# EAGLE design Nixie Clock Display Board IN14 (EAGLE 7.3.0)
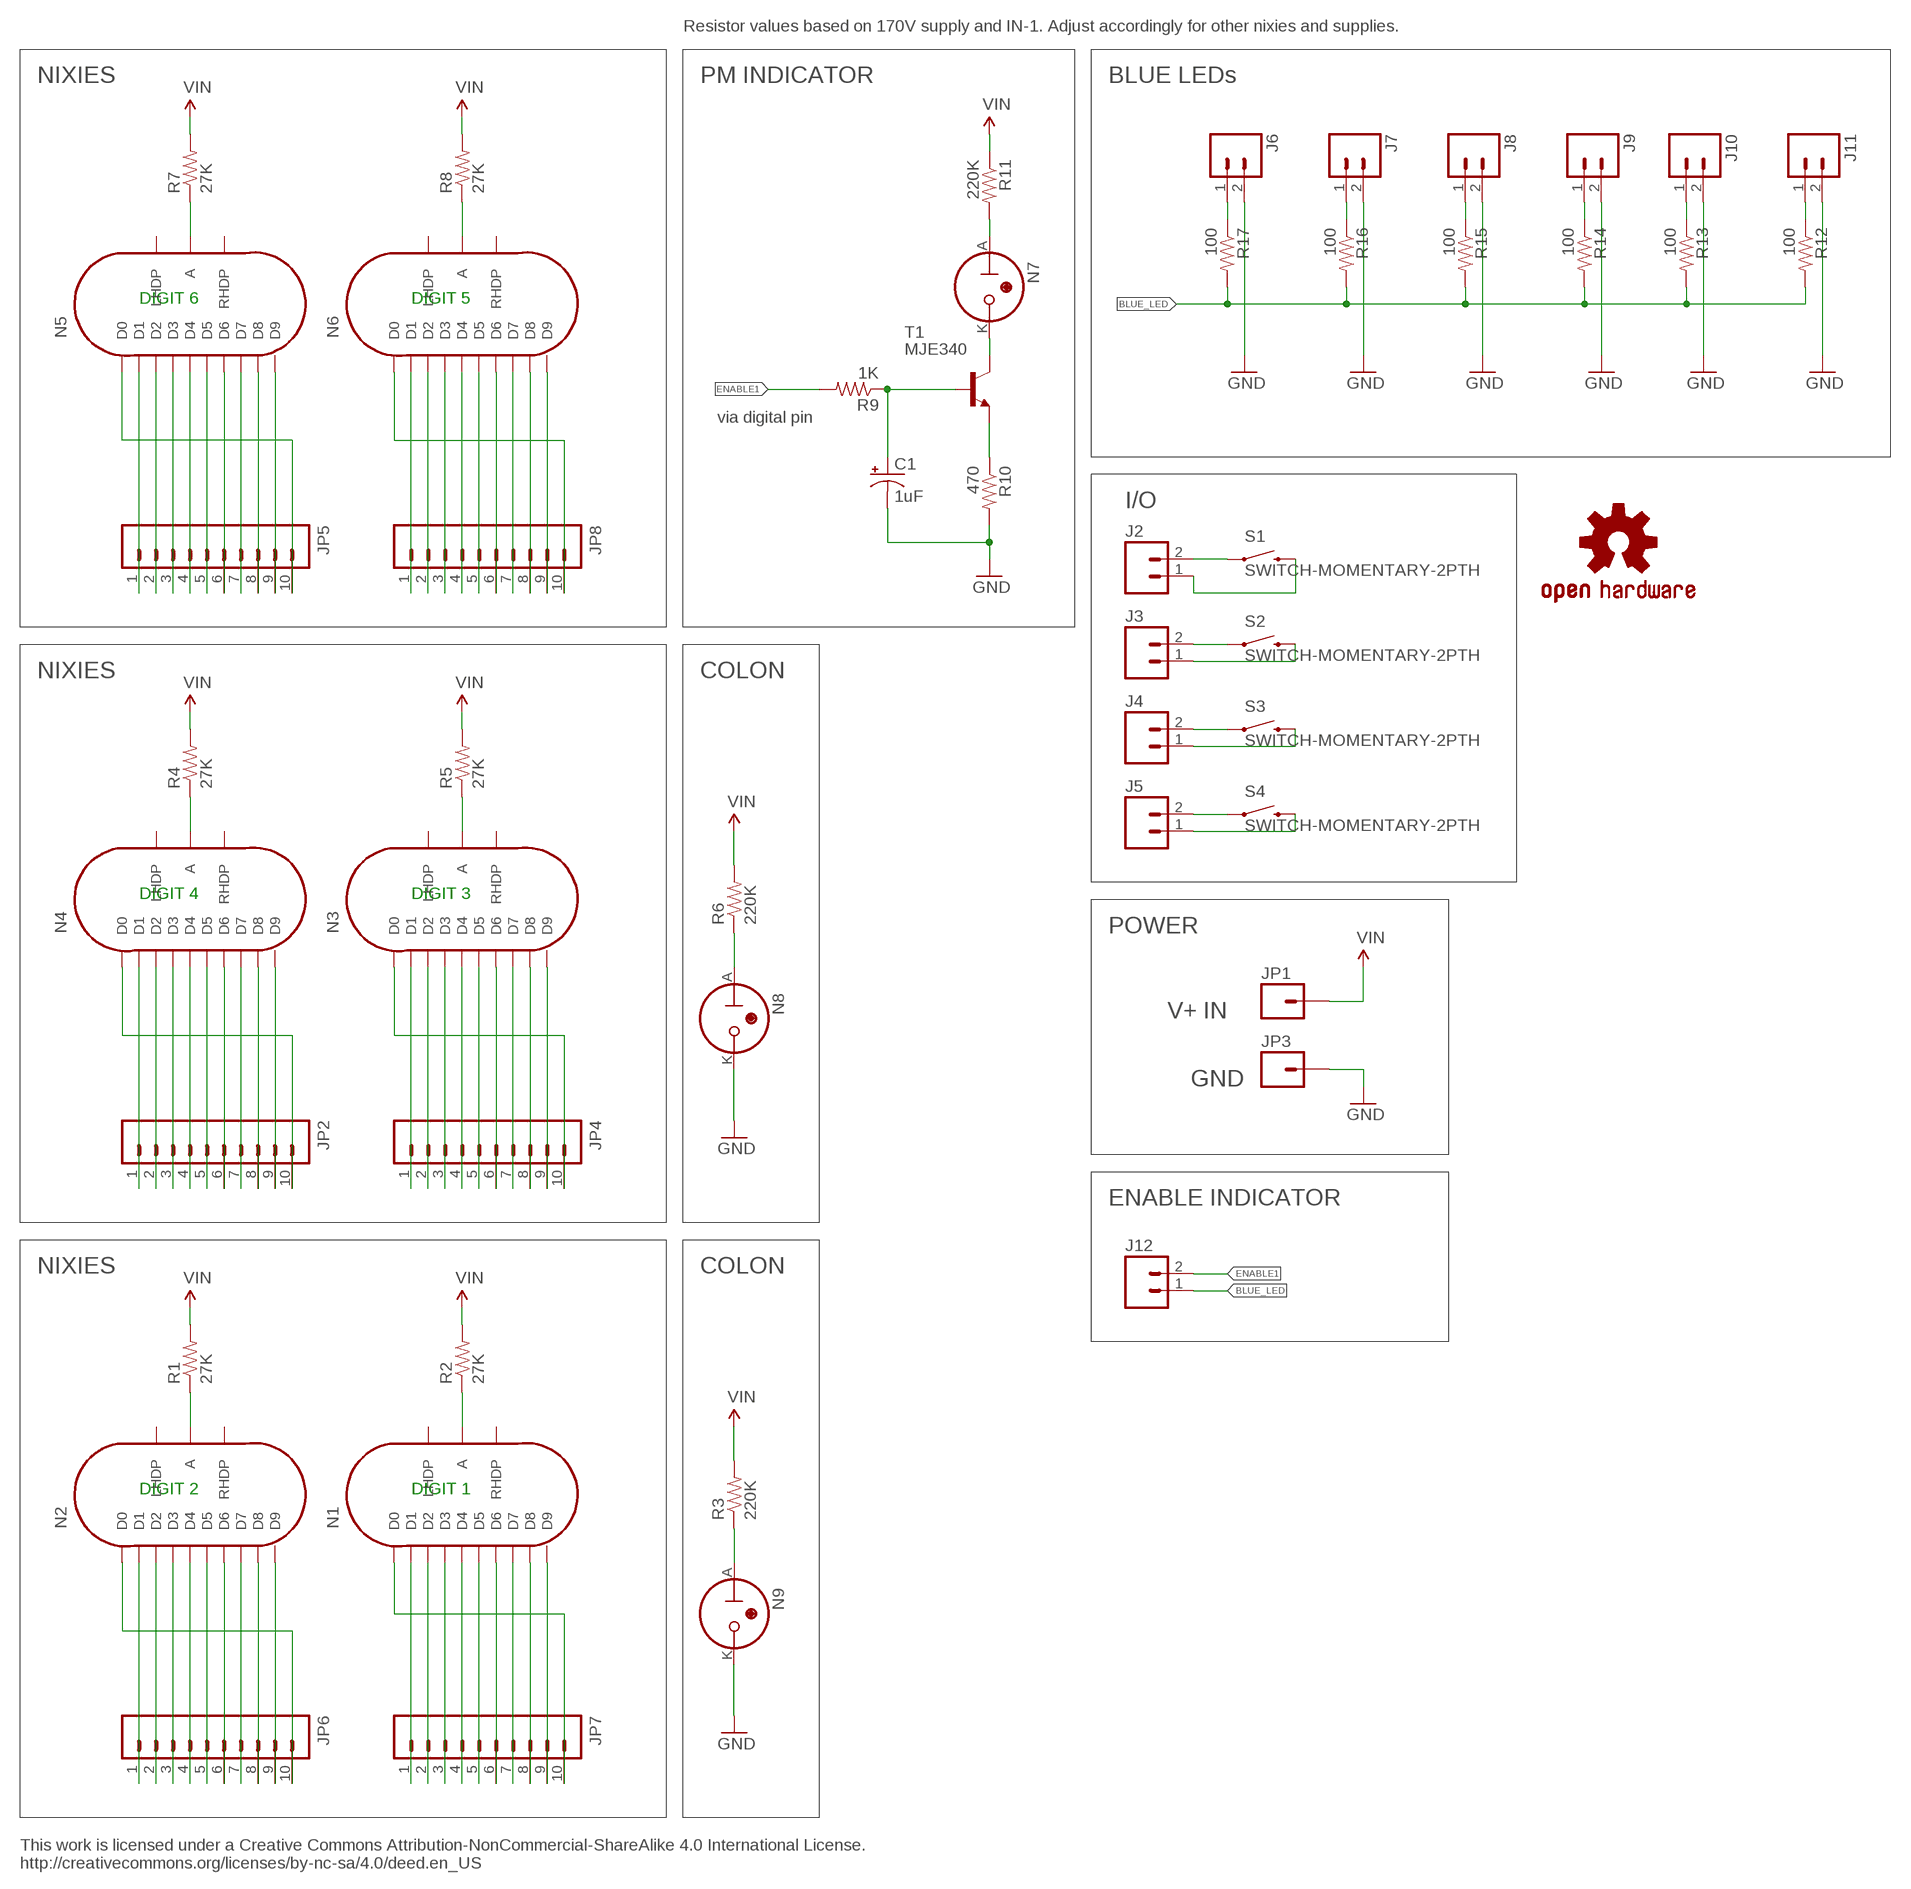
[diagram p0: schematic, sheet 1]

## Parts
C1  1uF  CAP_POLPTH2  [CPOL-RADIAL-10UF-25V]
J2  M02PTH  [1X02]
J3  M02PTH  [1X02]
J4  M02PTH  [1X02]
J5  M02PTH  [1X02]
J6  M02PTH  [1X02]
J7  M02PTH  [1X02]
J8  M02PTH  [1X02]
J9  M02PTH  [1X02]
J10  M02PTH  [1X02]
J11  M02PTH  [1X02]
J12  M02PTH  [1X02]
JP1  M01PTH  [1X01]
JP2  M10"  [1X10]
JP3  M01PTH  [1X01]
JP4  M10"  [1X10]
JP5  M10"  [1X10]
JP6  M10"  [1X10]
JP7  M10"  [1X10]
JP8  M10"  [1X10]
N1  IN-14  [IN-14]
N2  IN-14  [IN-14]
N3  IN-14  [IN-14]
N4  IN-14  [IN-14]
N5  IN-14  [IN-14]
N6  IN-14  [IN-14]
N7  IN-3  [IN-3]
N8  IN-3  [IN-3]
N9  IN-3  [IN-3]
R1  27K  RESISTORPTH-1/2W  [AXIAL-0.5]
R2  27K  RESISTORPTH-1/2W  [AXIAL-0.5]
R3  220K  RESISTORPTH-1/2W  [AXIAL-0.5]
R4  27K  RESISTORPTH-1/2W  [AXIAL-0.5]
R5  27K  RESISTORPTH-1/2W  [AXIAL-0.5]
R6  220K  RESISTORPTH-1/2W  [AXIAL-0.5]
R7  27K  RESISTORPTH-1/2W  [AXIAL-0.5]
R8  27K  RESISTORPTH-1/2W  [AXIAL-0.5]
R9  1K  RESISTORPTH-1/2W  [AXIAL-0.5]
R10  470  RESISTORPTH-1/2W  [AXIAL-0.5]
R11  220K  RESISTORPTH-1/2W  [AXIAL-0.5]
R12  100  RESISTOR0805-RES  [0805]
R13  100  RESISTOR0805-RES  [0805]
R14  100  RESISTOR0805-RES  [0805]
R15  100  RESISTOR0805-RES  [0805]
R16  100  RESISTOR0805-RES  [0805]
R17  100  RESISTOR0805-RES  [0805]
S1  SWITCH-MOMENTARY-2PTH  [TACTILE-PTH]
S2  SWITCH-MOMENTARY-2PTH  [TACTILE-PTH]
S3  SWITCH-MOMENTARY-2PTH  [TACTILE-PTH]
S4  SWITCH-MOMENTARY-2PTH  [TACTILE-PTH]
T1  MJE340  -NPN-TO225AA  [TO225AA]
U$2  OSHW-LOGOM  [OSHW-LOGO-M]

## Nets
BLUE_LED: J12.1 R12.2 R13.2 R14.2 R15.2 R16.2 R17.2
ENABLE1: J12.2 R9.P$2
GND: C1.2(-) J6.2 J7.2 J8.2 J9.2 J10.2 J11.2 JP3.1 N8.K N9.K R10.P$2
N$1: N8.A R6.P$1
N$4: J2.1 S1.3
N$5: J2.2 S1.1
N$6: J3.2 S2.1
N$7: JP2.6 N4.D6
N$8: JP2.9 N4.D9
N$9: JP2.8 N4.D8
N$10: JP2.10 N4.D0
N$11: JP2.7 N4.D7
N$12: JP2.5 N4.D5
N$13: JP2.4 N4.D4
N$14: JP2.3 N4.D3
N$15: JP2.2 N4.D2
N$16: JP2.1 N4.D1
N$17: JP4.6 N3.D6
N$18: JP4.9 N3.D9
N$19: JP4.8 N3.D8
N$20: JP4.10 N3.D0
N$21: J3.1 S2.3
N$22: C1.1(+) R9.P$1 T1.1(B)
N$23: N7.A R11.P$2
N$24: R10.P$1 T1.3(E)
N$25: JP4.7 N3.D7
N$26: JP4.5 N3.D5
N$27: J4.2 S3.1
N$28: N7.K T1.2(C)
N$29: N5.A R7.P$1
N$30: JP5.6 N5.D6
N$31: JP5.9 N5.D9
N$32: JP5.8 N5.D8
N$33: JP5.10 N5.D0
N$34: JP5.7 N5.D7
N$35: JP5.5 N5.D5
N$36: JP5.4 N5.D4
N$37: JP5.3 N5.D3
N$38: JP5.2 N5.D2
N$39: JP5.1 N5.D1
N$40: N6.A R8.P$1
N$41: JP8.6 N6.D6
N$42: JP8.9 N6.D9
N$43: JP8.8 N6.D8
N$44: JP8.10 N6.D0
N$45: JP8.7 N6.D7
N$46: JP8.5 N6.D5
N$47: JP8.4 N6.D4
N$48: JP8.3 N6.D3
N$49: JP8.2 N6.D2
N$50: JP8.1 N6.D1
N$51: JP4.4 N3.D4
N$52: JP4.3 N3.D3
N$53: JP4.2 N3.D2
N$54: JP4.1 N3.D1
N$55: N4.A R4.P$1
N$56: N3.A R5.P$1
N$57: N9.A R3.P$1
N$58: J4.1 S3.3
N$59: J5.2 S4.1
N$60: J5.1 S4.3
N$62: J6.1 R17.1
N$63: JP6.6 N2.D6
N$64: JP6.9 N2.D9
N$65: JP6.8 N2.D8
N$66: JP6.10 N2.D0
N$67: JP6.7 N2.D7
N$68: JP6.5 N2.D5
N$69: JP6.4 N2.D4
N$70: JP6.3 N2.D3
N$71: JP6.2 N2.D2
N$72: JP6.1 N2.D1
N$73: JP7.6 N1.D6
N$74: JP7.9 N1.D9
N$75: JP7.8 N1.D8
N$76: JP7.10 N1.D0
N$77: JP7.7 N1.D7
N$78: JP7.5 N1.D5
N$79: JP7.4 N1.D4
N$80: JP7.3 N1.D3
N$81: JP7.2 N1.D2
N$82: JP7.1 N1.D1
N$83: N2.A R1.P$1
N$84: N1.A R2.P$1
N$87: J7.1 R16.1
N$90: J8.1 R15.1
N$93: J9.1 R14.1
N$96: J10.1 R13.1
N$99: J11.1 R12.1
VIN: JP1.1 R1.P$2 R2.P$2 R3.P$2 R4.P$2 R5.P$2 R6.P$2 R7.P$2 R8.P$2 R11.P$1
Unconnected: N1.LHDP N1.RHDP N2.LHDP N2.RHDP N3.LHDP N3.RHDP N4.LHDP N4.RHDP N5.LHDP N5.RHDP N6.LHDP N6.RHDP

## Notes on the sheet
- Resistor values based on 170V supply and IN-1. Adjust accordingly for other nixies and supplies.
- NIXIES | PM INDICATOR | BLUE LEDs
- DIGIT 6 | DIGIT 5
- via digital pin
- I/O
- NIXIES | COLON
- DIGIT 4 | DIGIT 3
- POWER
- V+ IN
- GND
- ENABLE INDICATOR
- NIXIES | COLON
- DIGIT 2 | DIGIT 1
- This work is licensed under a Creative Commons Attribution-NonCommercial-ShareAlike 4.0 International License.
  http://creativecommons.org/licenses/by-nc-sa/4.0/deed.en_US

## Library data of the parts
C1 = SparkFun-Capacitors:CAP_POL: Capacitor Polarized
J2-J12 = SparkFun-Connectors:M02: Standard 2-pin 0.1" header. Use with
JP1 JP3 = SparkFun-Connectors:M01: Header 1
JP2 JP4-JP8 = SparkFun-Connectors:M10: Header 10 Standard 10-pin 0.1" header. Use with straight break away headers (SKU : PRT-00116), right angle break away headers (PRT-00553), swiss pins (PRT-00743), machine pins (PRT-00117), and female headers (PRT-00115).
N1-N6 = russian-nixies:IN-14: IN-14: medium numeric frontview nixie tube
N7-N9 = Nixie Tubes 2:IN-3: IN-3: nixie bulb
R1-R17 = SparkFun-Resistors:RESISTOR: Resistor
S1-S4 = SparkFun-Electromechanical:SWITCH-MOMENTARY-2: Various NO switches- pushbuttons, reed, etc; PROD_ID: SWCH-08441
T1 = Transistor 2:*-NPN-: NPN Transistror BF959 corrected 2008.03.06
U$2 = SparkFun:OSHW-LOGO: Open Source Hardware Logo This logo indicates the piece of hardware it is found on incorporates a OSHW license and/or adheres to the definition of open source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

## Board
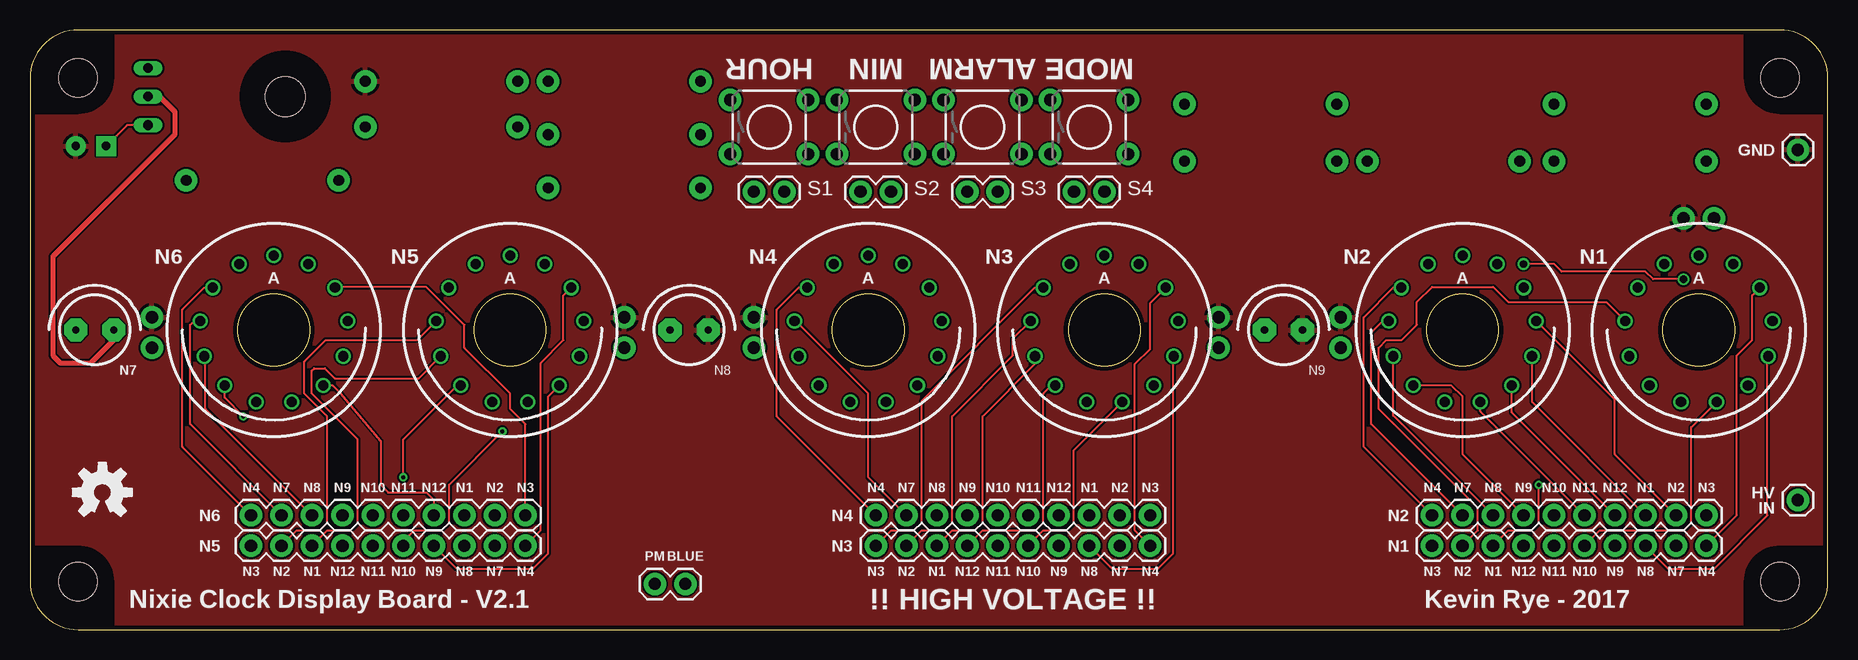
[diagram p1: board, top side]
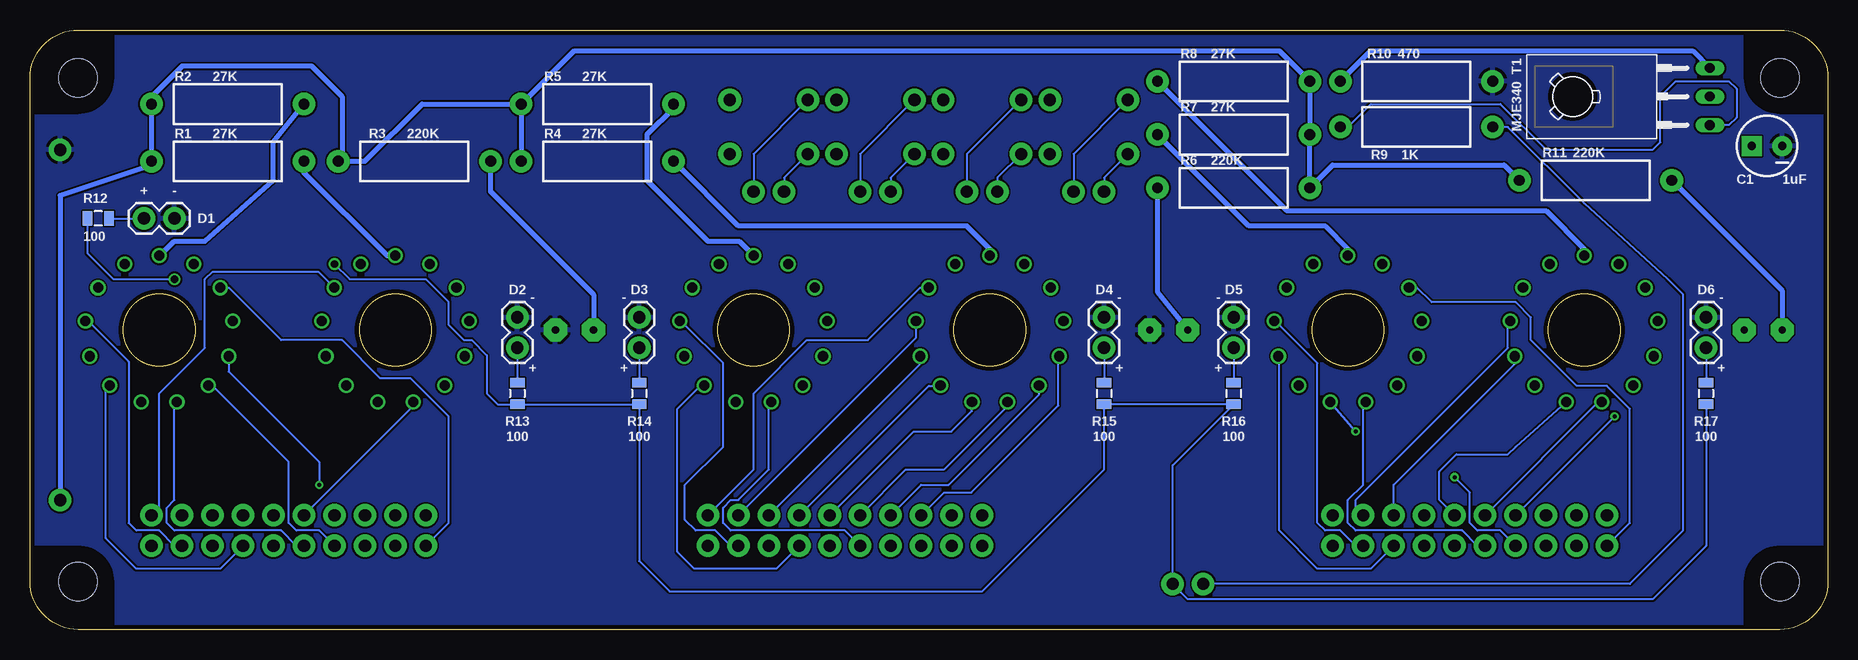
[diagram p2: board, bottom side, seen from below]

Size 149.83 x 50 mm. Coordinates in mm from the lower left corner, seen from the top.
Outline: circle at 20.32,24.99 radius 3
Outline: circle at 40.01,24.99 radius 3
Outline: circle at 69.85,24.99 radius 3
Outline: circle at 89.53,24.99 radius 3
Outline: circle at 119.38,24.99 radius 3
Outline: circle at 139.06,24.99 radius 3
Copper layers (1*16): Top 0.0356mm / dielectric 1.5011mm / Bottom 0.0356mm
Design rules "LaenPCBOrder": minimum track width 6mil, minimum drill 13mil, track to track 6mil, track to pad 6mil, pad to pad 6mil, via to via 6mil, smd to smd 6mil, copper to edge 15mil, drill to drill 6mil, minimum pad ring 7mil, minimum via ring 7mil, stop-mask expansion 3mil, vias tented up to drill 0mil, thermal gap 10mil

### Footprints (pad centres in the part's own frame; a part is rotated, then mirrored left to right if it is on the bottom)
CPOL-RADIAL-10UF-25V = drill 0.7 pad 1.651 square: 1 1.27,0 | drill 0.7 pad 1.651: 2 -1.27,0
1X02 = drill 1.016 pad 1.88: 1 0,0; 2 2.54,0
1X01 = drill 1.016 pad 1.88: 1 0,0
1X10 = drill 1.016 pad 1.88: 1 0,0; 2 2.54,0; 3 5.08,0; 4 7.62,0; 5 10.16,0; 6 12.7,0; 7 15.24,0; 8 17.78,0; 9 20.32,0; 10 22.86,0
IN-14 = drill 0.84: A 0,-6.19; D0 -5.094,-3.516; D1 5.094,-3.516; D2 6.145,-0.746; D3 5.788,2.195; D4 4.105,4.633; D5 1.481,6.01; D6 -1.481,6.01; D7 -4.105,4.633; D8 -5.788,2.195; D9 -6.145,-0.746; LHDP 2.877,-5.481; RHDP -2.877,-5.481
IN-3 = drill 0.6 pad 1.93 octagon: A -1.587,0; K 1.587,0
AXIAL-0.5 = drill 0.9 pad 1.88: P$1 -6.35,0; P$2 6.35,0
0805 = smd 0.8 x 1.2: 1 -0.9,0; 2 0.9,0
TACTILE-PTH = drill 1.016 pad 1.88: 1 -3.251,2.261; 2 3.251,2.261; 3 -3.251,-2.261; 4 3.251,-2.261
TO225AA = drill 0.813 long: 1 -2.381,-11.43; 2 0,-11.43; 3 2.381,-11.43 | hole 3.302: 0,0
50X150 = hole 3.2: 4,4; 145.83,4; 145.83,46; 4,46

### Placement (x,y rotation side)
C1  5.08,40.32 180 bottom
J2  60.33,36.51 0 top
J3  69.22,36.51 0 top
J4  78.11,36.51 0 top
J5  87,36.51 0 top
J6  10.16,23.5 90 bottom
J7  49.53,23.5 90 bottom
J8  60.33,23.5 90 bottom
J9  99.06,23.5 90 bottom
J10  109.22,23.5 90 bottom
J11  140.34,34.29 0 bottom
J12  54.61,3.81 180 top
JP1  147.32,10.79 0 top
JP2  70.48,9.53 0 top
JP3  147.32,40.01 0 top
JP4  70.48,6.99 0 top
JP5  18.41,6.99 0 top
JP6  116.84,9.53 0 top
JP7  116.84,6.99 0 top
JP8  18.41,9.53 0 top
N1  139.06,24.99 180 top
N2  119.38,24.99 180 top
N3  89.53,24.99 180 top
N4  69.85,24.99 180 top
N5  40.01,24.99 180 top
N6  20.32,24.99 180 top
N7  5.4,24.99 0 top
N8  54.93,24.99 0 top
N9  104.46,24.99 0 top
R1  133.35,39.05 180 bottom
R2  133.35,43.81 180 bottom
R3  117.79,39.05 180 bottom
R4  102.55,39.05 180 bottom
R5  102.55,43.81 180 bottom
R6  49.53,36.83 0 bottom
R7  49.53,41.27 0 bottom
R8  49.53,45.72 0 bottom
R9  34.29,41.91 0 bottom
R10  34.29,45.72 0 bottom
R11  19.37,37.47 0 bottom
R12  144.15,34.29 180 bottom
R13  109.22,19.68 270 bottom
R14  99.06,19.68 270 bottom
R15  60.33,19.68 270 bottom
R16  49.53,19.68 270 bottom
R17  10.16,19.68 270 bottom
S1  61.59,41.91 0 top
S2  70.48,41.91 0 top
S3  79.38,41.91 0 top
S4  88.27,41.91 0 top
T1  21.27,44.45 90 bottom
U$1  [50X150]  0,0 0 top
U$2  6.03,11.43 0 top

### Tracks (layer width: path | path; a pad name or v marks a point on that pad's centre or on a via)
BLUE_LED  (via drill 0.61)
  Top 0.152: v137.79,29.21 135.25,29.21 134.62,29.84 127.64,29.84 127,30.48 v124.46,30.48
  Bottom 0.152: R17.2 10.16,6.99 14.61,2.54 53.34,2.54 J12.1 54.61,13.71 R16.2 R15.2 60.33,13.34 70.48,3.17 96.52,3.17 99.06,5.71 R14.2 R13.2 110.86,18.79 111.76,19.68 111.76,22.86 113.03,24.13 113.67,24.13 114.94,25.4 114.94,27.3 116.84,29.21 123.19,29.21 v124.46,30.48 | R12.2 145.04,31.38 142.88,29.21 v137.79,29.21
ENABLE1
  Bottom 0.152: R9.P$2 26.67,41.91 20.32,35.56 13.34,29.21 12.06,27.94 12.06,8.26 16.51,3.81 J12.2
GND
  pour Bottom: -0.64,50.8 150.5,50.8 150.5,-0.64 -0.64,-0.64
  pour Top: -1.27,51.44 151.13,51.44 151.13,-1.27 -1.27,-1.27
N$1
  Bottom 0.406: R6.P$1 55.88,28.16 N8.A
N$4
  Bottom 0.152: S1.3 60.33,37.67 J2.1
N$5
  Bottom 0.152: S1.1 62.87,39.65 J2.2
N$6
  Bottom 0.152: S2.1 71.75,39.65 J3.2
N$7
  Bottom 0.152: JP2.6 76.2,16.51 73.04,16.51 71.33,18.22 N4.D6
N$8
  Bottom 0.152: JP2.9 76,24.34 N4.D9
N$9
  Bottom 0.152: JP2.8 75.64,22.15 N4.D8
N$10
  Bottom 0.152: JP2.10 89.53,13.34 89.53,19.68 85.09,24.13 80.01,24.13 75.64,28.5 N4.D0
N$11
  Bottom 0.152: JP2.7 74.93,20.32 74.3,20.32 N4.D7
N$12
  Bottom 0.152: JP2.5 76.83,13.34 73.66,13.34 68.37,18.63 N4.D5
N$13
  Bottom 0.152: JP2.4 75.56,12.06 73.28,12.06 65.75,19.6 N4.D4
N$14
  Bottom 0.152: JP2.3 73.66,11.43 71.38,11.43 64.14,18.67 64.14,22.23 N4.D3
N$15
  Top 0.152: JP2.2 69.85,12.7 69.85,19.68 63.8,25.73 N4.D2
N$16
  Top 0.152: JP2.1 62.23,17.78 62.23,26.67 64.06,28.5 N4.D1
N$17
  Top 0.152: JP4.6 84.45,8.26 86.36,8.26 87,8.89 87,14.96 N3.D6
N$18
  Bottom 0.152: JP4.9 91.44,6.99 92.71,8.26 94.35,8.26 95.25,9.15 95.25,12.06 92.08,15.24 92.08,22.23 95.25,25.4 N3.D9
N$19
  Top 0.152: JP4.8 90.17,5.08 93.98,5.08 95.25,6.35 95.25,22.72 N3.D8
N$20
  Top 0.152: JP4.10 92.08,8.26 92.08,22.14 93.34,23.41 93.34,27.22 N3.D0
N$21
  Bottom 0.152: S2.3 69.22,37.67 J3.1
N$22
  Top 0.152: T1.1 8.1,42.07 C1.1
  Bottom 0.152: R9.P$1 40.01,41.91 38.1,43.81 27.3,43.81 23.5,40.01 14.61,40.01 13.97,40.64 13.97,44.45 12.7,45.72 8.26,45.72 7.62,45.09 7.62,42.7 8.26,42.07 T1.1
N$23
  Bottom 0.406: R11.P$2 3.81,28.26 N7.A
N$24
  Bottom 0.406: R10.P$1 38.1,48.26 11.27,48.26 T1.3
N$25
  Bottom 0.152: JP4.7 87.63,5.08 94.47,5.08 95.89,6.5 95.89,18.41 93.98,20.32 N3.D7
N$26
  Bottom 0.152: JP4.5 81.92,8.26 91.44,8.26 92.08,8.89 92.08,10.16 91.44,10.79 90.81,10.79 88.27,13.34 88.27,18.41 N3.D5
N$27
  Bottom 0.152: S3.1 80.64,39.65 J4.2
N$28
  Top 0.406: T1.2 10.79,44.45 12.06,43.18 12.06,41.27 1.91,31.11 1.91,22.86 2.54,22.23 5.08,22.23 6.99,24.13 N7.K
N$29
  Bottom 0.406: N5.A 40.01,31.75 41.91,33.66 48.26,33.66 R7.P$1
N$30  (via drill 0.33)
  Top 0.152: v39.37,16.51 34.92,12.06 34.92,8.89 34.29,8.26 32.01,8.26 31.11,7.36 JP5.6
  Bottom 0.152: v39.37,16.51 N5.D6
N$31
  Bottom 0.152: JP5.9 39.37,6.99 40.64,8.26 41.91,8.26 42.55,8.89 42.55,22.23 45.72,25.4 N5.D9
N$32
  Bottom 0.152: JP5.8 38.1,5.08 42.55,5.08 45.72,8.26 45.72,22.23 N5.D8
N$33
  Top 0.152: JP5.10 42.55,8.26 42.55,22.23 44.45,24.13 44.45,27.85 N5.D0
N$34
  Top 0.152: JP5.7 35.56,5.08 41.91,5.08 43.18,6.35 43.18,19.42 N5.D7
N$35
  Bottom 0.152: JP5.5 29.21,6.99 30.48,8.26 39.37,8.26 40.01,8.89 40.01,10.79 38.73,12.06 38.73,18.41 N5.D5
N$36  (via drill 0.33)
  Top 0.152: v31.11,12.7 31.11,15.88 35.59,20.35 N5.D4
  Bottom 0.152: v31.11,12.7 29.84,11.43 29.84,8.89 29.21,8.26 27.3,8.26 JP5.4
N$37
  Top 0.152: JP5.3 24.77,8.26 26.67,8.26 27.3,8.89 27.3,15.88 23.5,19.68 23.5,21.59 23.68,21.78 24.58,21.78 25.4,20.95 32.38,20.95 N5.D3
N$38
  Top 0.152: JP5.2 22.23,8.26 24.13,8.26 24.77,8.89 24.77,17.78 22.86,19.68 22.86,22.33 24.66,24.13 32.26,24.13 N5.D2
N$39
  Bottom 0.152: JP5.1 16.51,8.89 16.51,18.41 18.41,20.32 20.95,20.32 24.77,24.13 24.77,26.04 26.04,27.3 33.02,27.3 34.29,28.57 N5.D1
N$40
  Bottom 0.406: N6.A 20.32,31.75 23.5,34.92 45.09,34.92 R8.P$1
N$41
  Bottom 0.152: JP8.6 32.38,10.79 32.38,13.19 30.96,14.61 26.67,14.61 26.04,15.24 N6.D6
N$42
  Bottom 0.152: JP8.9 39.37,9.53 39.37,10.79 26.67,23.5 26.67,25.4 N6.D9
N$43
  Bottom 0.152: JP8.8 36.2,12.06 26.04,22.23 N6.D8
N$44
  Top 0.152: JP8.10 41.27,17.14 40.01,18.41 40.01,19.68 36.2,23.5 36.2,25.4 33.02,28.57 26.04,28.57 N6.D0
N$45
  Top 0.152: JP8.7 33.66,10.79 33.02,11.43 29.84,11.43 29.21,12.06 29.21,15.74 25.9,19.68 25.23,20.35 N6.D7
N$46
  Bottom 0.152: JP8.5 19.12,18.98 N6.D5
N$47  (via drill 0.33)
  Top 0.152: v17.78,17.78 16.21,19.34 N6.D4
  Bottom 0.152: JP8.4 v17.78,17.78
N$48
  Top 0.152: JP8.3 14.61,18.41 14.61,22.23 N6.D3
N$49
  Top 0.152: JP8.2 13.34,17.14 13.34,25.4 13.67,25.73 N6.D2
N$50
  Top 0.152: JP8.1 12.7,15.24 12.7,26.67 14.53,28.5 N6.D1
N$51
  Top 0.152: JP4.4 79.38,8.26 83.82,8.26 84.45,8.89 84.45,19.68 85.12,20.35 N3.D4
N$52
  Top 0.152: JP4.3 76.83,8.26 78.74,8.26 79.38,8.89 79.38,17.78 83.75,22.15 N3.D3
N$53
  Top 0.152: JP4.2 74.3,8.26 76.2,8.26 76.83,8.89 76.83,17.78 81.92,22.86 81.92,24.26 N3.D2
N$54
  Top 0.152: JP4.1 71.75,8.26 73.66,8.26 74.3,8.89 74.3,19.05 83.75,28.5 N3.D1
N$55
  Bottom 0.406: N4.A 69.85,31.75 71.75,33.66 90.81,33.66 R4.P$1
N$56
  Bottom 0.406: R5.P$1 96.2,43.5 98.42,41.27 98.42,37.47 93.34,32.38 90.74,32.38 N3.A
N$57
  Bottom 0.406: N9.A 102.87,27.94 111.44,36.51 R3.P$1
N$58
  Bottom 0.152: S3.3 78.11,37.67 J4.1
N$59
  Bottom 0.152: S4.1 89.53,39.65 J5.2
N$60
  Bottom 0.152: S4.3 87,37.67 J5.1
N$62
  Bottom 0.152: J6.1 R17.1
N$63
  Top 0.152: JP6.6 120.86,18.2 N2.D6
N$64
  Top 0.152: JP6.9 132.08,14.61 132.08,19.18 N2.D9
N$65
  Top 0.152: JP6.8 125.17,18.98 N2.D8
N$66
  Bottom 0.152: JP6.10 139.06,10.16 139.06,19.68 135.25,23.5 135.25,29.21 134.62,29.84 125.82,29.84 N2.D0
N$67
  Top 0.152: JP6.7 123.48,18.12 N2.D7
N$68
  Bottom 0.152: JP6.5 117.9,18.63 N2.D5
N$69
  Top 0.152: JP6.4 119.38,14.61 119.38,19.42 118.45,20.35 N2.D4
N$70
  Top 0.152: JP6.3 113.59,17.85 N2.D3
N$71
  Top 0.152: JP6.2 111.76,17.14 111.76,24.77 112.73,25.73 N2.D2
N$72
  Top 0.152: JP6.1 111.12,15.24 111.12,26.04 113.59,28.5 N2.D1
N$73
  Top 0.152: JP7.6 130.81,8.26 137.79,8.26 138.43,8.89 138.43,16.86 N1.D6
N$74
  Bottom 0.152: N1.D9 144.99,25.73 141.6,22.35 141.6,8.89 140.97,8.26 139.06,8.26 137.79,6.99 JP7.9
N$75
  Top 0.152: JP7.8 136.53,5.08 140.34,5.08 144.78,9.53 144.78,22.72 N1.D8
N$76
  Top 0.152: JP7.10 142.24,9.53 142.24,22.86 143.51,24.13 143.51,27.85 N1.D0
N$77
  Bottom 0.152: JP7.7 133.99,5.08 140.97,5.08 143.51,7.62 143.51,20.01 N1.D7
N$78
  Bottom 0.152: JP7.5 127.64,6.99 128.91,8.26 137.79,8.26 138.43,8.89 138.43,10.16 137.79,10.79 137.79,18.77 N1.D5
N$79
  Bottom 0.152: JP7.4 125.73,8.26 127.64,8.26 128.27,8.89 128.27,13.97 134.65,20.35 N1.D4
N$80  (via drill 0.33)
  Top 0.152: v125.73,12.06 125.73,8.89 125.09,8.26 123.19,8.26 JP7.3
  Bottom 0.152: N1.D3 133.28,21.52 125.73,13.97 v125.73,12.06
N$81
  Top 0.152: JP7.2 120.65,8.26 120.65,10.16 112.39,18.41 112.39,23.5 113.03,24.13 114.3,24.13 115.57,25.4 115.57,27.3 116.84,28.57 121.92,28.57 123.19,27.3 131.35,27.3 N1.D2
N$82
  Bottom 0.152: JP7.1 114.94,8.89 114.94,17.78 118.11,20.95 120.65,20.95 123.83,24.13 128.91,24.13 133.28,28.5 N1.D1
N$83
  Bottom 0.406: N2.A 120.08,31.18 127,38.1 R1.P$1
N$84
  Bottom 0.406: N1.A 139,31.18 137.79,32.38 135.25,32.38 129.54,37.47 129.54,40.64 R2.P$1
N$87
  Bottom 0.152: J7.1 R16.1
N$90
  Bottom 0.152: J8.1 R15.1
N$93
  Bottom 0.152: J9.1 R14.1
N$96
  Bottom 0.152: J10.1 R13.1
N$99
  Bottom 0.152: R12.1 J11.1
VIN
  Bottom 0.406: JP1.1 147.32,36.2 139.7,38.73 R1.P$2 R2.P$2 139.7,44.45 137.16,46.99 126.36,46.99 123.83,44.45 123.83,39.37 R3.P$2 121.92,39.05 117.16,43.81 R5.P$2 | R5.P$2 R4.P$2 | R5.P$2 104.46,48.26 45.72,48.26 R8.P$2 R7.P$2 R6.P$2 41.27,38.73 26.99,38.73 R11.P$1

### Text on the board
Unrouted: This work is licensed under a Creative Commons Attribution-NonCommercial-ShareAlike 4.0 International License. / http://creativecommons.org/licenses/by-nc-sa/4.0/deed.en_US
tNames: HOUR | MIN | ALARM | MODE | GND | A | A | A | A | A | A | N4 | N7 | N8 | N9 | N10 | N11 | N12 | N1 | N2 | N3 | N4 | N7 | N8 | N9 | N10 | N11 | N12 | N1 | N2 | N3 | N4 | N7 | N8 | N9 | N10 | N11 | N12 | N1 | N2 | N3 | HV | N6 | N4 | N2 | IN | N5 | N3 | N1 | PM | BLUE | N3 | N2 | N1 | N12 | N11 | N10 | N9 | N8 | N7 | N4 | N3 | N2 | N1 | N12 | N11 | N10 | N9 | N8 | N7 | N4 | N3 | N2 | N1 | N12 | N11 | N10 | N9 | N8 | N7 | N4 | Nixie Clock Display Board - V2.1 | !! HIGH VOLTAGE !! | Kevin Rye - 2017
bNames: - | + | D1 | D6 | D5 | D4 | D3 | D2 | - | - | - | - | - | + | + | + | + | +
